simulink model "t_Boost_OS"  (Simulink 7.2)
settings: Solver=ode3  SolverMode=SingleTasking  StartTime=0.0  StopTime=0.01  FixedStep=10e-6  MaxStep=5e-6  RelTol=1e-6  AbsTol=1e-6

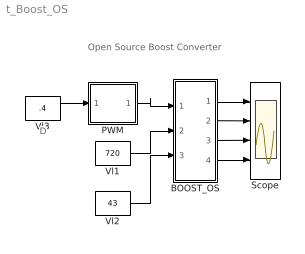
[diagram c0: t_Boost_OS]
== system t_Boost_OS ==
  note: Open Source Boost Converter
  note: D
  BOOST_OS : Subsystem  mask{L1=10e-3, IL0=40, C1=1e-3, UC0=1200, R1=1e5}
      mask prompts: L1 "Inductance L1"; IL0 "Initial Current"; C1 "Capacitance"; UC0 "Initial Voltage"; R1 "Load Resistance"
      mask help: Open Source boost Converter Input Vector u: u[0]= T1.gate u[1]= E.v u[2]= IDC.i Output Vector y: y[0]= T1.I y[1]= D1.I y[2]= L1.I y[3]= C1.V Parameter Vector p: p[0]= L1.L p[1]= L1.iL0 p[2]= C1.C p[3]= C1.vC0 p[4]= R1.r You can pause the simulation during running, change the Parameters you want and continue the Simulation
  PWM : Subsystem  mask(PWMtr){FS=1e3}
      mask prompts: FS "Frequency"
  Scope : Scope  NumInputPorts=4
  Vl1 : Constant  Value=720
  Vl2 : Constant  Value=43
  Vl3 : Constant  Value=.4
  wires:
  Vl3/1 -> PWM/1(In1)
  BOOST_OS/1(iT1) -> Scope/1
  BOOST_OS/2(iD1) -> Scope/2
  BOOST_OS/3(iL1) -> Scope/3
  BOOST_OS/4(vC) -> Scope/4
  PWM/1(Out1) -> BOOST_OS/1(sw)
  Vl1/1 -> BOOST_OS/2(E)
  Vl2/1 -> BOOST_OS/3(IDC)

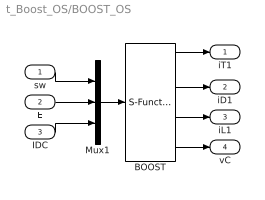
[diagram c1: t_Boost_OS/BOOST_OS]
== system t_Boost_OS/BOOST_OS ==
  sw : Inport  OutDataType=sfix(16)  OutScaling=2^0
  E : Inport  Port=2  OutDataType=sfix(16)  OutScaling=2^0
  IDC : Inport  Port=3  OutDataType=sfix(16)  OutScaling=2^0
  BOOST : S-Function  FunctionName=s_boost_OS  Parameters="[L1  IL0  C1   UC0  R1]"  EnableBusSupport=off
  Mux1 : Mux  Inputs=3
  iT1 : Outport  OutDataType=sfix(16)  OutScaling=2^0
  iD1 : Outport  Port=2  OutDataType=sfix(16)  OutScaling=2^0
  iL1 : Outport  Port=3  OutDataType=sfix(16)  OutScaling=2^0
  vC : Outport  Port=4  OutDataType=sfix(16)  OutScaling=2^0
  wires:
  Mux1/1 -> BOOST/1
  sw/1 -> Mux1/1
  E/1 -> Mux1/2
  BOOST/1 -> iT1/1
  BOOST/2 -> iD1/1
  BOOST/3 -> iL1/1
  BOOST/4 -> vC/1
  IDC/1 -> Mux1/3

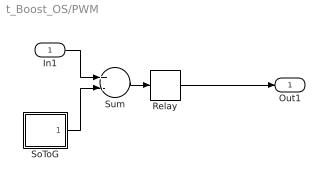
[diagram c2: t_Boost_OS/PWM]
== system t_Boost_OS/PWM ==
  In1 : Inport  OutDataType=sfix(16)  OutScaling=2^0
  Relay : Relay  OutDataType=sfix(16)  OutScaling=2^0
  SoToG : Subsystem  mask(SoToG){T=1/FS}
      mask prompts: T "Period Time"
  Sum : Sum  Inputs=+-  OutDataType=sfix(16)  OutScaling=2^0
  Out1 : Outport  InitialOutput=0
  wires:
  Sum/1 -> Relay/1
  In1/1 -> Sum/1
  SoToG/1(O) -> Sum/2
  Relay/1 -> Out1/1

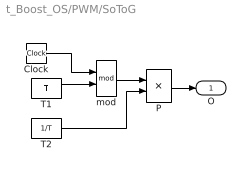
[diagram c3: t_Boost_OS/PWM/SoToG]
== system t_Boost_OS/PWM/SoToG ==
  Clock : Clock
  P : Product  OutDataType=sfix(16)  OutScaling=2^0
  T1 : Constant  Value=T  OutDataType=sfix(16)  OutScaling=2^0
  T2 : Constant  Value=1/T  OutDataType=sfix(16)  OutScaling=2^0
  mod : Math  Operator=mod
  O : Outport
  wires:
  Clock/1 -> mod/1
  T1/1 -> mod/2
  T2/1 -> P/2
  mod/1 -> P/1
  P/1 -> O/1
